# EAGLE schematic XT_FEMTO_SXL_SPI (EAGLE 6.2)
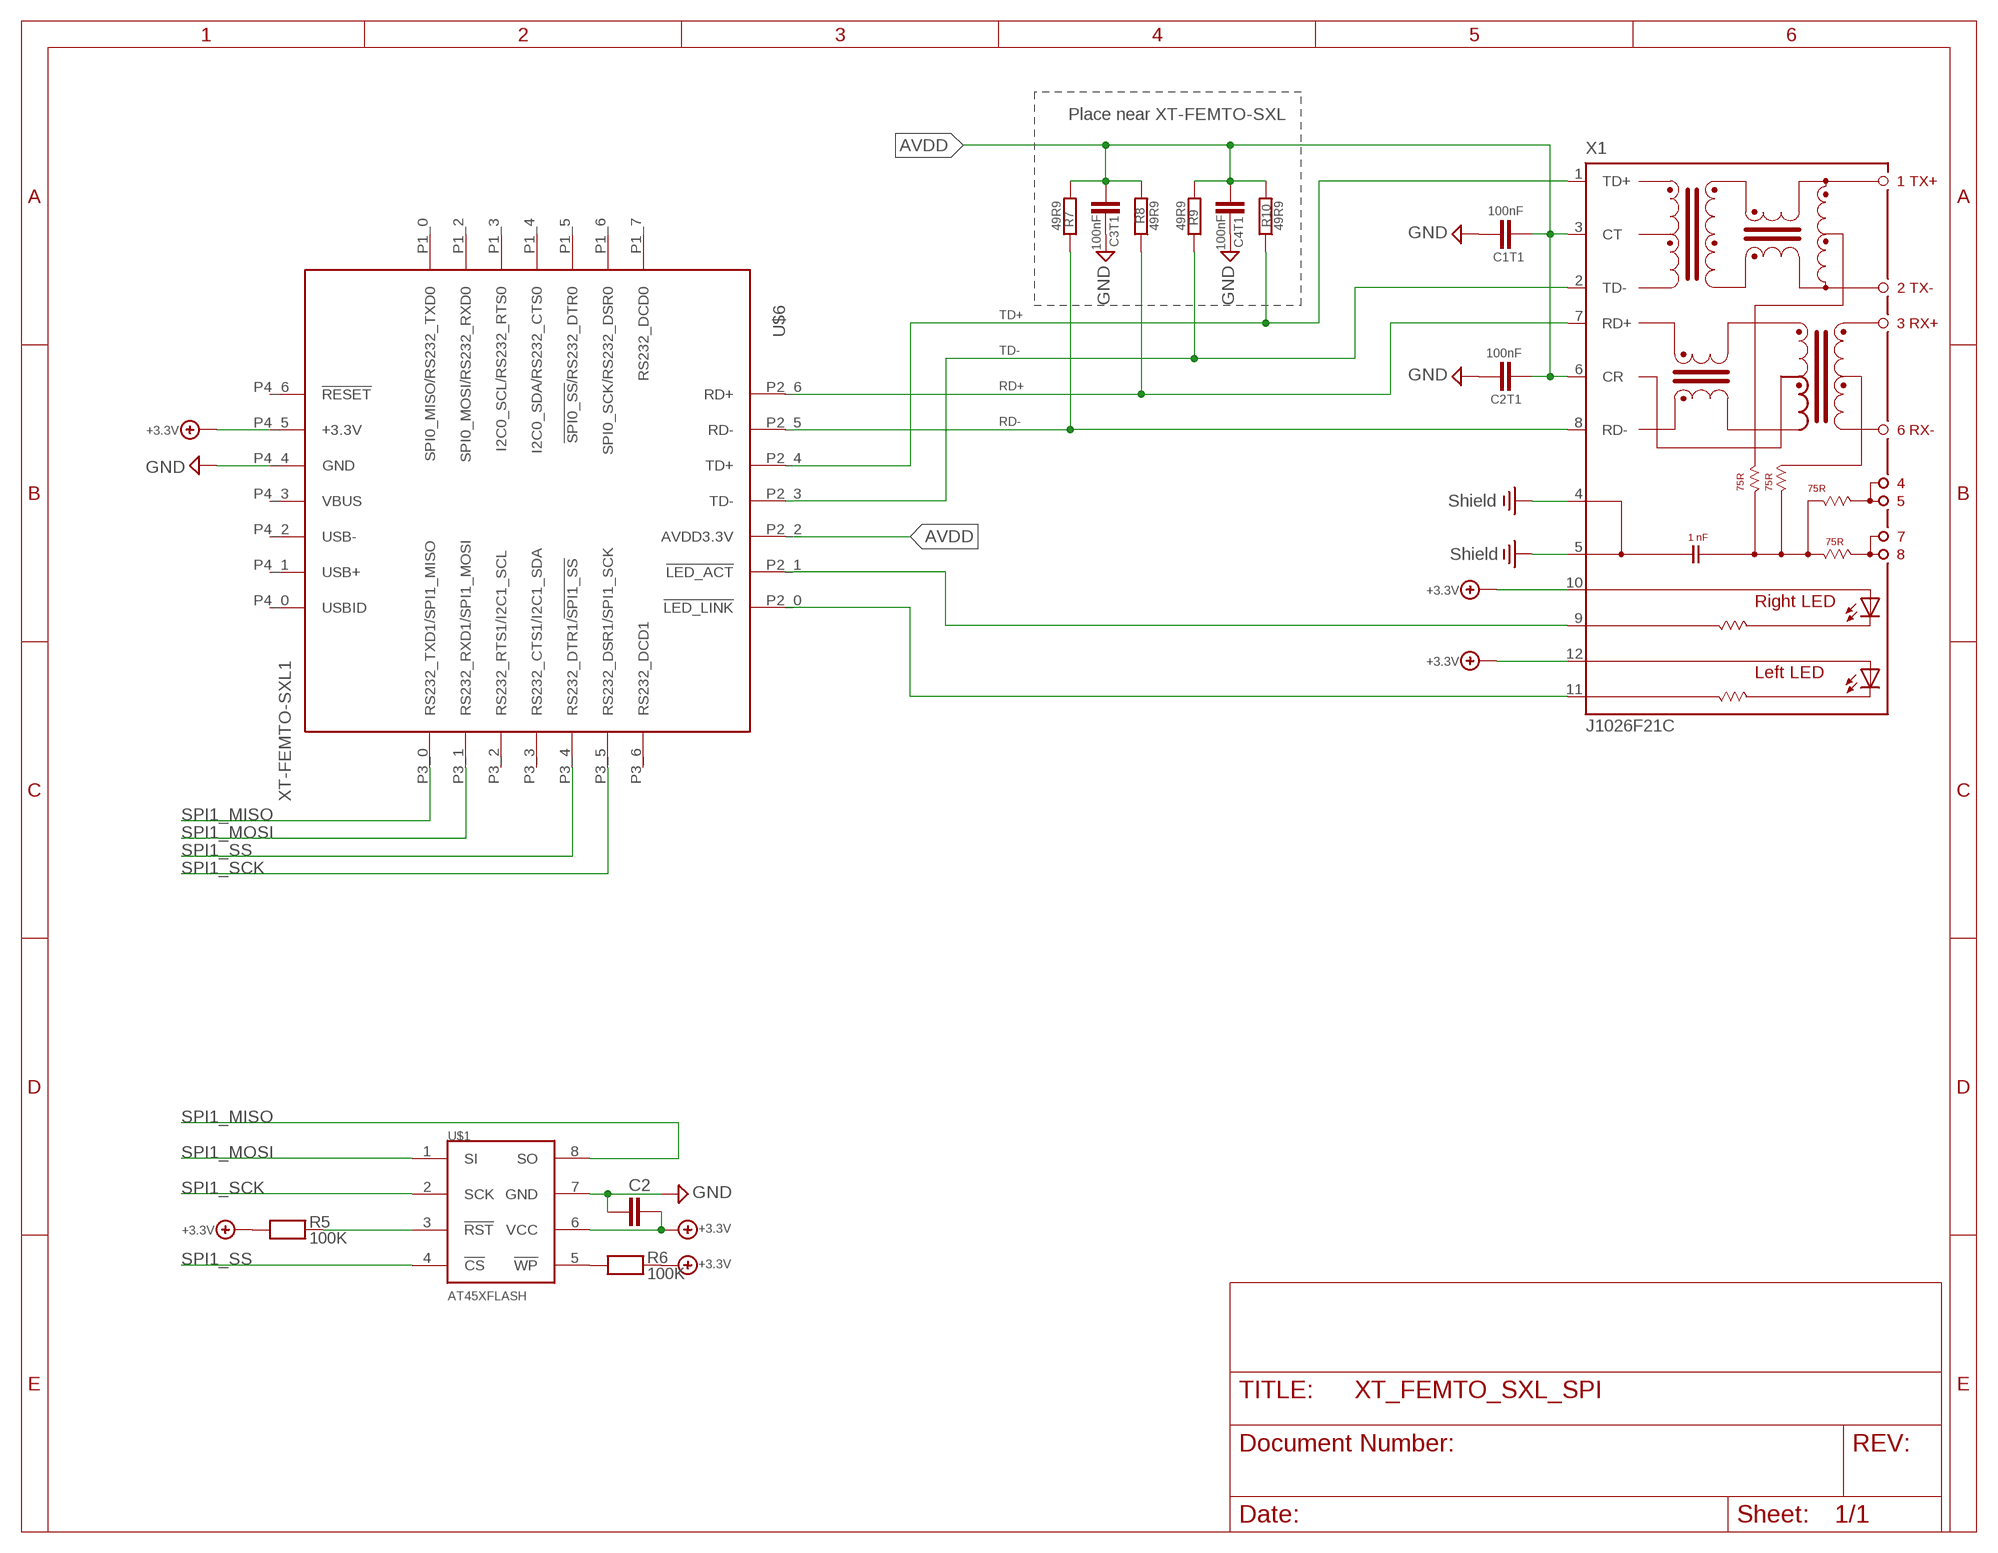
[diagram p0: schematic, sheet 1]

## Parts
C1T1  100nF  CHIP-C-VTS0402  [R0402_VTS]
C2  CHIP-C-0805  [SMD-0805]
C2T1  100nF  CHIP-C-VTS0402  [R0402_VTS]
C3T1  100nF  CHIP-C-VTS0402  [R0402_VTS]
C4T1  100nF  CHIP-C-VTS0402  [R0402_VTS]
R5  100K  CHIP-R-0603  [SMD-0603]
R6  100K  CHIP-R-0603  [SMD-0603]
R7  49R9  R-EU_R0603  [R0603]
R8  49R9  R-EU_R0603  [R0603]
R9  49R9  R-EU_R0603  [R0603]
R10  49R9  R-EU_R0603  [R0603]
U$1  AT45XFLASH  [SO-8]
U$6  XT-FEMTO-SXL1  [XT-FEMTO-SXL-PIN]
X1  J1026F21C  [J1]

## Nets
+3.3V: C2.2 R5.1 R6.2 U$1.6(VCC) U$6.P4_5(+3.3V) X1.10(A-R) X1.12(A-L)
AVDD: C1T1.1 C2T1.2 C3T1.1 C4T1.2 R7.2 R8.2 R9.2 R10.2 U$6.P2_2(AVDD3.3V) X1.3(CT) X1.6(CR)
GND: C1T1.2 C2.1 C2T1.1 C3T1.2 C4T1.1 U$1.7(GND) U$6.P4_4(GND)
N$3: R5.2 U$1.3(!RST)
N$5: R6.1 U$1.5(!WP)
N$7: U$6.P2_1(!LED_ACT) X1.9(C-R)
N$8: U$6.P2_0(!LED_LINK) X1.11(C-L)
PE: X1.4 X1.5 ; supply symbol labelled Shield
RD+: R8.1 U$6.P2_6(RD+) X1.7(RD+)
RD-: R7.1 U$6.P2_5(RD-) X1.8(RD-)
SPI1_MISO: U$1.8(SO) U$6.P3_0(RS232_TXD1/SPI1_MISO)
SPI1_MOSI: U$1.1(SI) U$6.P3_1(RS232_RXD1/SPI1_MOSI)
SPI1_SCK: U$1.2(SCK) U$6.P3_5(RS232_DSR1/SPI1_SCK)
SPI1_SS: U$1.4(!CS) U$6.P3_4(RS232_DTR1/!SPI1_SS!)
TD+: R10.1 U$6.P2_4(TD+) X1.1(TD+)
TD-: R9.1 U$6.P2_3(TD-) X1.2(TD-)
Unconnected: U$6.P1_0(SPI0_MISO/RS232_TXD0) U$6.P1_2(SPI0_MOSI/RS232_RXD0) U$6.P1_3(I2C0_SCL/RS232_RTS0) U$6.P1_4(I2C0_SDA/RS232_CTS0) U$6.P1_5(!SPI0_SS!/RS232_DTR0) U$6.P1_6(SPI0_SCK/RS232_DSR0) U$6.P1_7(RS232_DCD0) U$6.P3_2(RS232_RTS1/I2C1_SCL) U$6.P3_3(RS232_CTS1/I2C1_SDA) U$6.P3_6(RS232_DCD1) U$6.P4_0(USBID) U$6.P4_1(USB+) U$6.P4_2(USB-) U$6.P4_3(VBUS) U$6.P4_6(!RESET)

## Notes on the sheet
- Place near XT-FEMTO-SXL

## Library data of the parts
C1T1 C2T1 C3T1 C4T1 = mea-lib:CHIP-C-?: Chip capacitance
C2 = XTMACRO:CHIP-C-?: Chip capacitance
R5 R6 = XTMACRO:CHIP-R-?: Chip resistors
R7-R10 = rcl:R-EU_: RESISTOR, European symbol
U$1 = xtnano:AT45XFLASH
U$6 = ak-devices:XT-FEMTO-SXL: AK-NORD XT-FEMTO-SXL
X1 = con-pulse:J1026F: PULSEJACK (TM) 1x1 Tab-UP RJ45 10/100 Base-TX RJ45 1x1 Tab-UP with LEDs 8-pin (J1 series) and 6-pin (JP series) integrated magnetics connector, designed to support applications, such as ADSL modems, LAN-on-Motherboard, and Hub and Switches. Source: www.pulseeng.com .. PulseJack-J402.pdf; OC_FARNELL: unknown; OC_NEWARK: unknown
